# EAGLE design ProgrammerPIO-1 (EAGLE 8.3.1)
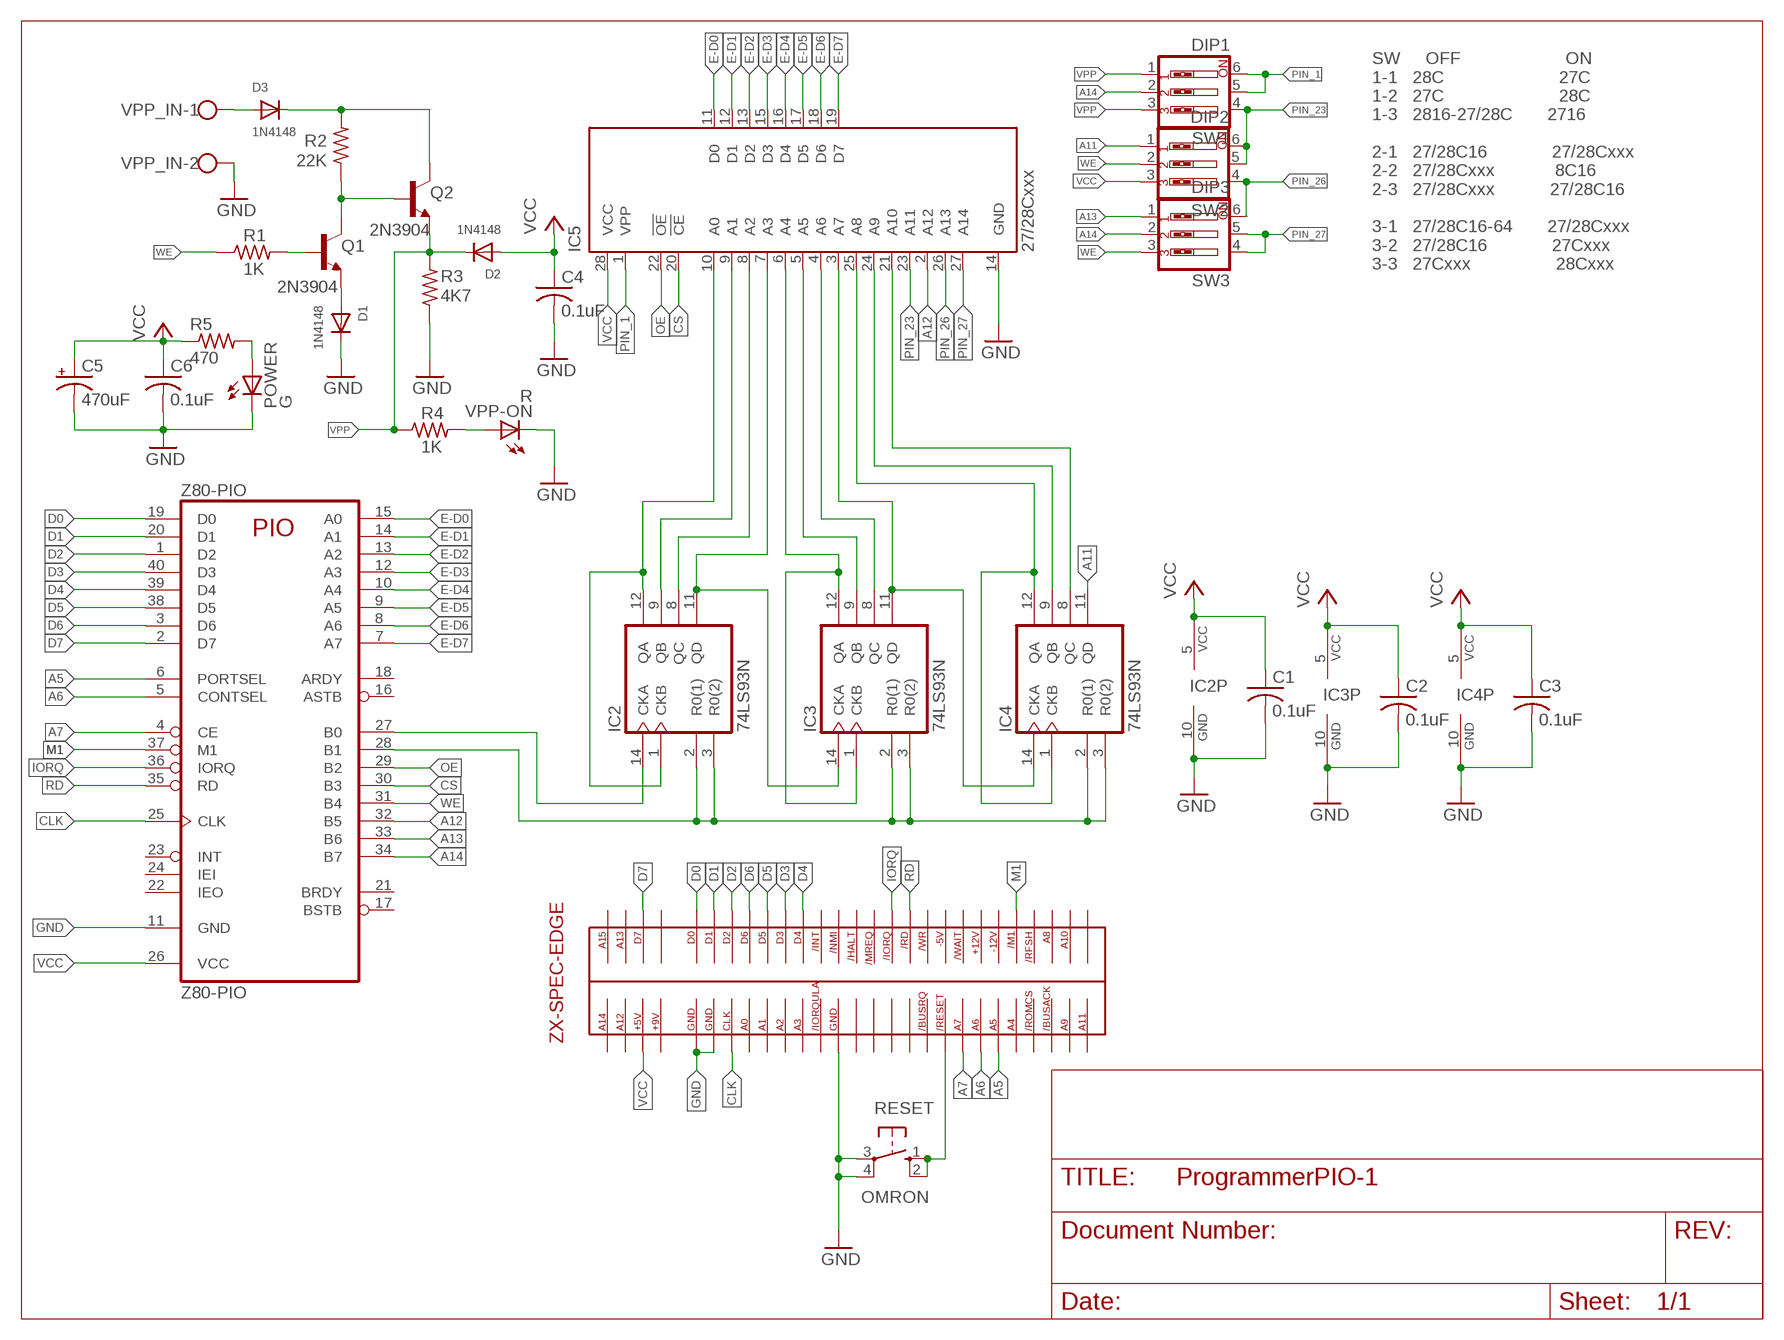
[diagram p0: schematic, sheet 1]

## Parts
1  ZX-EDGE-SPECCY  [ZX-EDGE-SPEC]
C1  0.1uF  C-US025-025X050  [C025-025X050]
C2  0.1uF  C-US025-025X050  [C025-025X050]
C3  0.1uF  C-US025-025X050  [C025-025X050]
C4  0.1uF  C-US025-025X050  [C025-025X050]
C5  470uF  CPOL-USE2.5-5  [E2,5-5]
C6  0.1uF  C-US025-025X050  [C025-025X050]
D1  1N4148  DIODEDO-1N4148  [DO-1N4148]
D2  1N4148  DIODEDO-1N4148  [DO-1N4148]
D3  1N4148  DIODEDO-1N4148  [DO-1N4148]
IC2  74LS93N  [DIL14]
IC3  74LS93N  [DIL14]
IC4  74LS93N  [DIL14]
IC5  27/28Cxxx  27C256P  [DIL28-6]
POWER  G  LED5MM  [LED5MM]
Q1  2N3904  [TO92]
Q2  2N3904  [TO92]
R1  1K  R-US_0204/7  [0204/7]
R2  22K  R-US_0204/7  [0204/7]
R3  4K7  R-US_0204/7  [0204/7]
R4  1K  R-US_0204/7  [0204/7]
R5  470  R-US_0204/7  [0204/7]
RESET  OMRON  10-XX  [B3F-10XX]
SW1  DIP1  SW_DIP-3  [EDG-03]
SW2  DIP2  SW_DIP-3  [EDG-03]
SW3  DIP3  SW_DIP-3  [EDG-03]
VPP-ON  R  LED5MM  [LED5MM]
VPP_IN  W237-102  [W237-102]
Z80-PIO  Z80-PIO  Z80PIO  [DIL40]

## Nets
A5: 1.A5 Z80-PIO.6(PORTSEL)
A6: 1.A6 Z80-PIO.5(CONTSEL)
A7: 1.A7 Z80-PIO.4(CE)
A11: IC4.11(QD) SW2.1
A12: IC5.2(A12) Z80-PIO.32(B5)
A13: SW3.1 Z80-PIO.33(B6)
A14: SW1.2 SW3.2 Z80-PIO.34(B7)
B0: IC2.14(CKA) Z80-PIO.27(B0)
B1: IC2.2(R0(1)) IC2.3(R0(2)) IC3.2(R0(1)) IC3.3(R0(2)) IC4.2(R0(1)) IC4.3(R0(2)) Z80-PIO.28(B1)
CLK: 1.CLK Z80-PIO.25(CLK)
CS: IC5.20(!CE) Z80-PIO.30(B3)
D0: 1.D0 Z80-PIO.19(D0)
D1: 1.D1 Z80-PIO.20(D1)
D2: 1.D2 Z80-PIO.1(D2)
D3: 1.D3 Z80-PIO.40(D3)
D4: 1.D4 Z80-PIO.39(D4)
D5: 1.D5 Z80-PIO.38(D5)
D6: 1.D6 Z80-PIO.3(D6)
D7: 1.D7 Z80-PIO.2(D7)
E-D0: IC5.11(D0) Z80-PIO.15(A0)
E-D1: IC5.12(D1) Z80-PIO.14(A1)
E-D2: IC5.13(D2) Z80-PIO.13(A2)
E-D3: IC5.15(D3) Z80-PIO.12(A3)
E-D4: IC5.16(D4) Z80-PIO.10(A4)
E-D5: IC5.17(D5) Z80-PIO.9(A5)
E-D6: IC5.18(D6) Z80-PIO.8(A6)
E-D7: IC5.19(D7) Z80-PIO.7(A7)
GND: 1.GND1 1.GND2 1.GND3 C1.2 C2.2 C3.2 C4.2 C5.- C6.2 D1.C IC2.10(GND) IC3.10(GND) IC4.10(GND) IC5.14(GND) POWER.K(C) R3.1 RESET.3(P) RESET.4(P1) VPP-ON.K(C) VPP_IN.2 Z80-PIO.11(GND)
IORQ: 1./IORQ Z80-PIO.36(IORQ)
M1: 1./M1 Z80-PIO.37(M1)
N$1: IC2.1(CKB) IC2.12(QA) IC5.10(A0)
N$2: IC2.9(QB) IC5.9(A1)
N$3: IC2.8(QC) IC5.8(A2)
N$4: IC2.11(QD) IC3.14(CKA) IC5.7(A3)
N$5: IC3.1(CKB) IC3.12(QA) IC5.6(A4)
N$6: IC3.9(QB) IC5.5(A5)
N$7: IC3.8(QC) IC5.4(A6)
N$8: IC3.11(QD) IC4.14(CKA) IC5.3(A7)
N$9: IC4.1(CKB) IC4.12(QA) IC5.25(A8)
N$10: IC4.9(QB) IC5.24(A9)
N$11: IC4.8(QC) IC5.21(A10)
N$13: Q1.2(B) R1.2
N$14: D1.A Q1.3(E)
N$15: Q1.1(C) Q2.2(B) R2.1
N$16: D3.A VPP_IN.1
N$17: D3.C Q2.1(C) R2.2
N$18: R4.2 VPP-ON.A
N$19: 1./RST RESET.1(S) RESET.2(S1)
N$20: POWER.A R5.2
OE: IC5.22(!OE) Z80-PIO.29(B2)
PIN_1: IC5.1(VPP) SW1.5 SW1.6
PIN_23: IC5.23(A11) SW1.4 SW2.5 SW2.6
PIN_26: IC5.26(A13) SW2.4 SW3.6
PIN_27: IC5.27(A14) SW3.4 SW3.5
RD: 1./RD Z80-PIO.35(RD)
VCC: 1.+5 C1.1 C2.1 C3.1 C4.1 C5.+ C6.1 D2.A IC2.5(VCC) IC3.5(VCC) IC4.5(VCC) IC5.28(VCC) R5.1 SW2.3 Z80-PIO.26(VCC)
VPP: D2.C Q2.3(E) R3.2 R4.1 SW1.1 SW1.3
WE: R1.1 SW2.2 SW3.3 Z80-PIO.31(B4)
Unconnected: 1.+9 1.+12 1.-5(-5V) 1.-12 1./BUSAK 1./BUSRQ 1./HALT 1./INT 1./IORQULA 1./MREQ 1./NMI 1./RFSH(/REFSH) 1./ROMCS 1./WAIT 1./WR 1.A0 1.A1 1.A2 1.A3 1.A4 1.A8 1.A9 1.A10 1.A11 1.A12 1.A13 1.A14 1.A15 1.N/C1 1.N/C2 1.N/C3 1.N/C4 1.N/C5 1.N/C6 Z80-PIO.16(ASTB) Z80-PIO.17(BSTB) Z80-PIO.18(ARDY) Z80-PIO.21(BRDY) Z80-PIO.22(IEO) Z80-PIO.23(INT) Z80-PIO.24(IEI)

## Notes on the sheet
- SW     OFF                     ON
  1-1   28C                       27C
  1-2   27C                       28C
  1-3   2816-27/28C       2716
  
  2-1   27/28C16             27/28Cxxx
  2-2   27/28Cxxx            8C16
  2-3   27/28Cxxx           27/28C16
  
  3-1   27/28C16-64       27/28Cxxx
  3-2   27/28C16             27Cxxx
  3-3   27Cxxx                 28Cxxx

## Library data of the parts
1 = sinclair-zx-spec:ZX-EDGE-SPECCY: ZX SPECTRUM EDGE CONNECTOR
C1-C4 C6 = rcl:C-US: CAPACITOR, American symbol
C5 = rcl:CPOL-US: POLARIZED CAPACITOR, American symbol
D1-D3 = adafruit:DIODE: Diode
IC2-IC4 = 74xx-us:74*93: Decade, divide by twelve and binary COUNTER
IC5 = microchip:27*256: CMOS EPROM 256 K (32 K x 8), low voltage; MF: Arrow Electronics; MPN: M27C256B15F1; OC_FARNELL: 1125431; OC_NEWARK: 93K7335
POWER = adafruit:LED: LED
Q1 Q2 = transistor-npn:2N3904: NPN Transistor
R1-R5 = rcl:R-US_: RESISTOR, American symbol
RESET = switch-omron:10-XX: OMRON SWITCH; MPN: B3F-1000; OC_FARNELL: 176432; OC_NEWARK: 36M3542
SW1-SW3 = special:SW_DIP-3: DIP SWITCH
VPP-ON = led:LED: LED
VPP_IN = con-wago-500:W237-102: WAGO SCREW CLAMP; MPN: 237-102; OC_FARNELL: unknown; OC_NEWARK: 70K9898
Z80-PIO = zilog:Z80PIO: Z80 FAMILY DEVICE

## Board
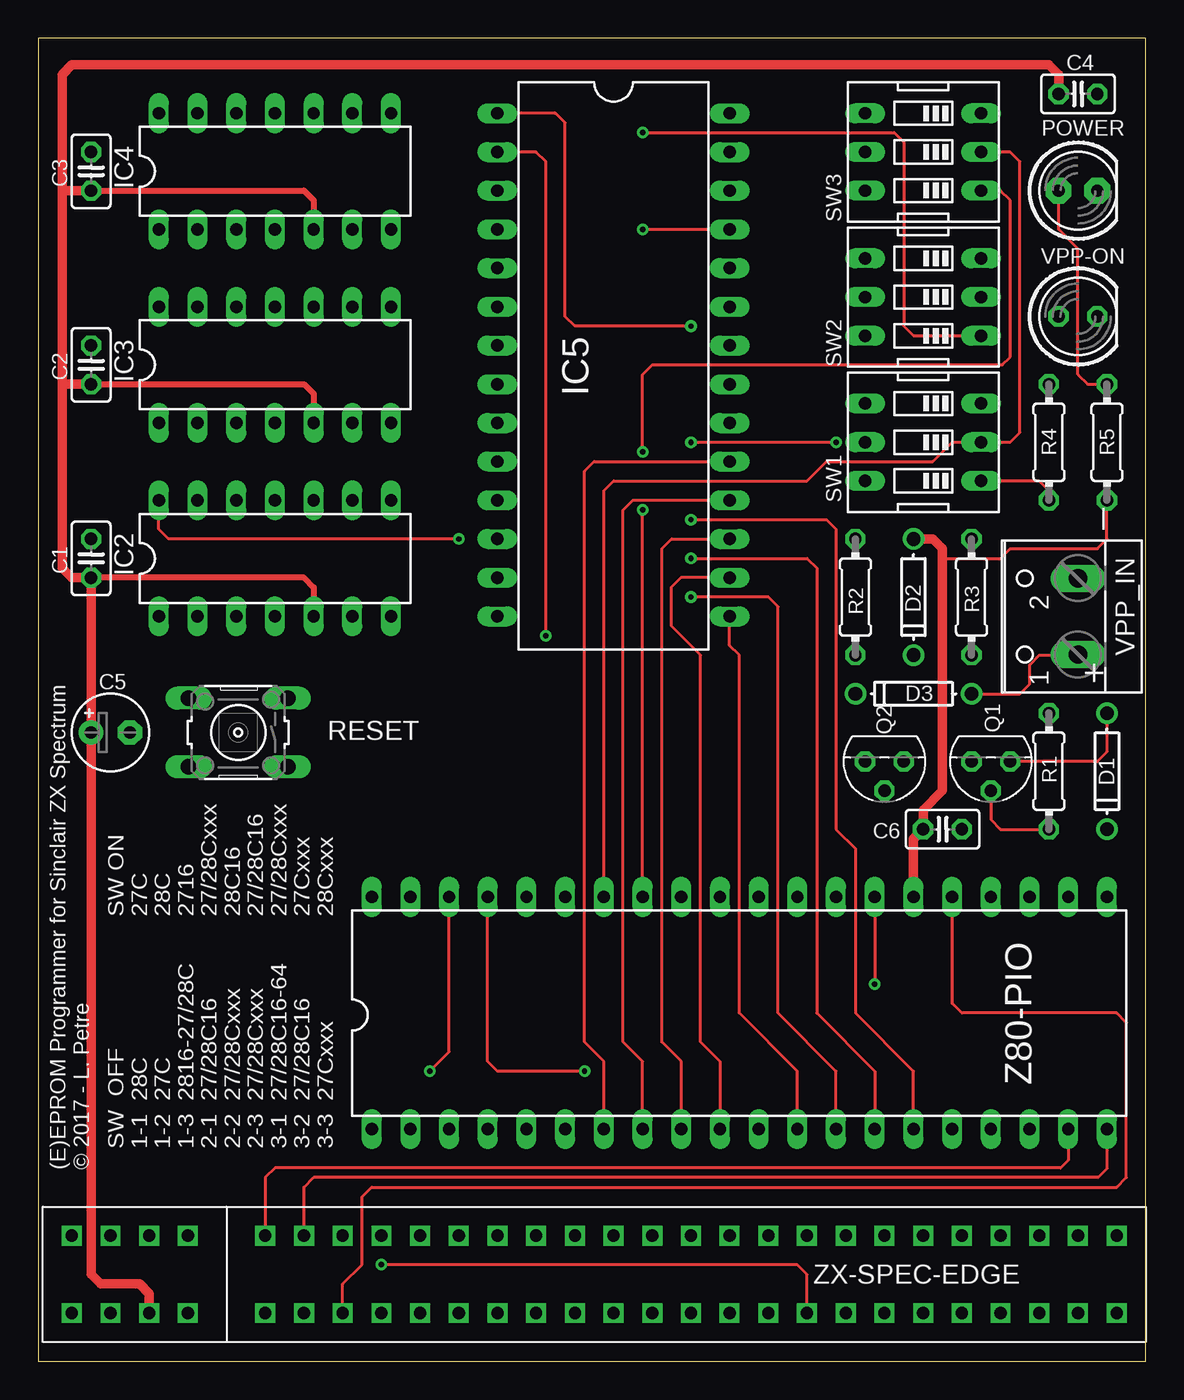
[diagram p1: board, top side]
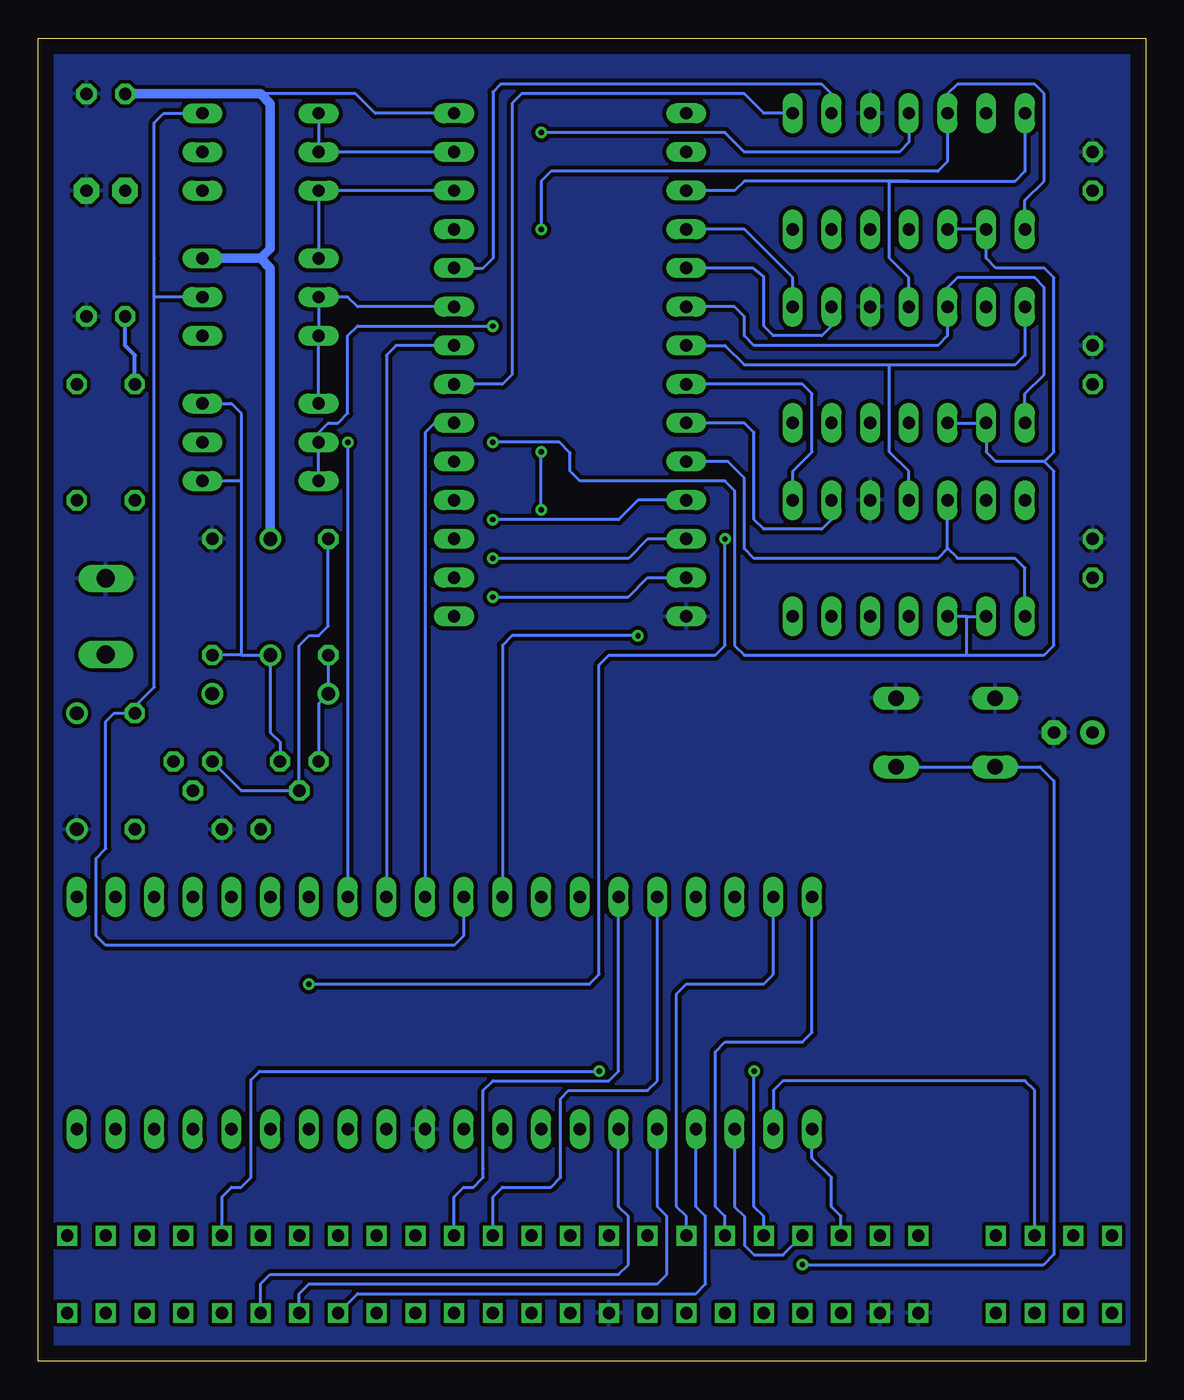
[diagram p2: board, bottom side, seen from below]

Size 72.7 x 86.85 mm. Coordinates in mm from the lower left corner, seen from the top.
Outline: 72.7,0 72.7,86.85 0,86.85 0,0 72.7,0
Copper layers (1*16): Top 0.035mm / dielectric 1.5mm / Bottom 0.035mm
Design rules "default": minimum track width 6mil, minimum drill 0.35mm, track to track 6mil, track to pad 6mil, pad to pad 6mil, via to via 6mil, smd to smd 6mil, copper to edge 40mil, drill to drill 6mil, minimum pad ring 10mil, minimum via ring 8mil, stop-mask expansion 4mil, vias tented up to drill 0mil, thermal gap 10mil

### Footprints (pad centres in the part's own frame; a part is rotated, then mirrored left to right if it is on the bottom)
ZX-EDGE-SPEC = drill 0.8 square: +5 -5.08,-2.54; +9 -2.54,-2.54; +12 43.18,2.54; -5 38.1,2.54; -12 45.72,2.54; /BUSAK 53.34,-2.54; /BUSRQ 35.56,-2.54; /HALT 25.4,2.54; /INT 20.32,2.54; /IORQ 30.48,2.54; /IORQULA 20.32,-2.54; /M1 48.26,2.54; /MREQ 27.94,2.54; /NMI 22.86,2.54; /RD 33.02,2.54; /RFSH 50.8,2.54; /ROMCS 50.8,-2.54; /RST 38.1,-2.54; /WAIT 40.64,2.54; /WR 35.56,2.54; A0 10.16,-2.54; A1 12.7,-2.54; A2 15.24,-2.54; A3 17.78,-2.54; A4 48.26,-2.54; A5 45.72,-2.54; A6 43.18,-2.54; A7 40.64,-2.54; A8 53.34,2.54; A9 55.88,-2.54; A10 55.88,2.54; A11 58.42,-2.54; A12 -7.62,-2.54; A13 -7.62,2.54; A14 -10.16,-2.54; A15 -10.16,2.54; CLK 7.62,-2.54; D0 2.54,2.54; D1 5.08,2.54; D2 7.62,2.54; D3 15.24,2.54; D4 17.78,2.54; D5 12.7,2.54; D6 10.16,2.54; D7 -5.08,2.54; GND1 2.54,-2.54; GND2 5.08,-2.54; GND3 22.86,-2.54; N/C1 -2.54,2.54; N/C2 58.42,2.54; N/C3 25.4,-2.54; N/C4 27.94,-2.54; N/C5 30.48,-2.54; N/C6 33.02,-2.54
C025-025X050 = drill 0.813 octagon: 1 -1.27,0; 2 1.27,0
E2,5-5 = drill 0.813 pad 1.6: + -1.27,0 | drill 0.813 pad 1.6 octagon: - 1.27,0
DO-1N4148 = drill 0.9: A -3.81,0; C 3.81,0
DIL14 = drill 0.813 long: 1 -7.62,-3.81; 2 -5.08,-3.81; 3 -2.54,-3.81; 4 0,-3.81; 5 2.54,-3.81; 6 5.08,-3.81; 7 7.62,-3.81; 8 7.62,3.81; 9 5.08,3.81; 10 2.54,3.81; 11 0,3.81; 12 -2.54,3.81; 13 -5.08,3.81; 14 -7.62,3.81
DIL28-6 = drill 0.813 long: 1 -16.51,-7.62; 2 -13.97,-7.62; 3 -11.43,-7.62; 4 -8.89,-7.62; 5 -6.35,-7.62; 6 -3.81,-7.62; 7 -1.27,-7.62; 8 1.27,-7.62; 9 3.81,-7.62; 10 6.35,-7.62; 11 8.89,-7.62; 12 11.43,-7.62; 13 13.97,-7.62; 14 16.51,-7.62; 15 16.51,7.62; 16 13.97,7.62; 17 11.43,7.62; 18 8.89,7.62; 19 6.35,7.62; 20 3.81,7.62; 21 1.27,7.62; 22 -1.27,7.62; 23 -3.81,7.62; 24 -6.35,7.62; 25 -8.89,7.62; 26 -11.43,7.62; 27 -13.97,7.62; 28 -16.51,7.62
LED5MM = drill 0.813 pad 1.676 octagon: A -1.27,0; K 1.27,0
TO92 = drill 0.813 octagon: 1 1.27,0; 2 0,1.905; 3 -1.27,0
0204/7 = drill 0.813 octagon: 1 -3.81,0; 2 3.81,0
B3F-10XX = drill 1.016 long: 1 -3.251,2.261; 2 3.251,2.261; 3 -3.251,-2.261; 4 3.251,-2.261
EDG-03 = drill 0.813 long: 1 -2.54,-3.81; 2 0,-3.81; 3 2.54,-3.81; 4 2.54,3.81; 5 0,3.81; 6 -2.54,3.81
LED5MM' = drill 0.813 octagon: A -1.27,0; K 1.27,0
W237-102 = drill 1.194 long: 1 -2.5,-1.27; 2 2.5,-1.27
DIL40 = drill 0.813 long: 1 -24.13,-7.62; 2 -21.59,-7.62; 3 -19.05,-7.62; 4 -16.51,-7.62; 5 -13.97,-7.62; 6 -11.43,-7.62; 7 -8.89,-7.62; 8 -6.35,-7.62; 9 -3.81,-7.62; 10 -1.27,-7.62; 11 1.27,-7.62; 12 3.81,-7.62; 13 6.35,-7.62; 14 8.89,-7.62; 15 11.43,-7.62; 16 13.97,-7.62; 17 16.51,-7.62; 18 19.05,-7.62; 19 21.59,-7.62; 20 24.13,-7.62; 21 24.13,7.62; 22 21.59,7.62; 23 19.05,7.62; 24 16.51,7.62; 25 13.97,7.62; 26 11.43,7.62; 27 8.89,7.62; 28 6.35,7.62; 29 3.81,7.62; 30 1.27,7.62; 31 -1.27,7.62; 32 -3.81,7.62; 33 -6.35,7.62; 34 -8.89,7.62; 35 -11.43,7.62; 36 -13.97,7.62; 37 -16.51,7.62; 38 -19.05,7.62; 39 -21.59,7.62; 40 -24.13,7.62

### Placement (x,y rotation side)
1  12.37,5.71 0 top
C1  3.48,52.7 90 top
C2  3.48,65.41 90 top
C3  3.48,78.11 90 top
C4  68.25,83.19 0 top
C5  4.75,41.27 0 top
C6  59.36,34.92 0 top
D1  70.16,38.73 270 top
D2  57.45,50.16 270 top
D3  57.45,43.81 180 top
IC2  15.54,52.7 0 top
IC3  15.54,65.41 0 top
IC4  15.54,78.11 0 top
IC5  37.77,65.41 270 top
POWER  68.25,76.83 0 top
Q1  62.54,39.37 180 top
Q2  55.55,39.37 180 top
R1  66.34,38.73 270 top
R2  53.65,50.16 270 top
R3  61.27,50.16 270 top
R4  66.34,60.33 90 top
R5  70.16,60.33 90 top
RESET  13.13,41.27 180 top
SW1  58.09,60.33 90 top
SW2  58.09,69.85 90 top
SW3  58.09,79.38 90 top
VPP-ON  R  [LED5MM']  68.25,68.58 0 top
VPP_IN  66.98,48.9 90 top
Z80-PIO  46.02,22.86 0 top

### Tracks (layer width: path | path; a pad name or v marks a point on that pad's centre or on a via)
A5
  Bottom 0.2: 1.A5 58.09,5.08 57.45,5.71 34.59,5.71 33.96,6.35 33.96,9.53 34.59,10.16 Z80-PIO.6
A6
  Bottom 0.2: 1.A6 55.55,4.45 54.91,5.08 32.05,5.08 31.42,5.71 31.42,9.53 32.05,10.16 Z80-PIO.5
A7
  Bottom 0.2: 1.A7 51.74,4.45 29.52,4.45 28.88,5.08 28.88,9.53 29.52,10.16 Z80-PIO.4
A11  (via drill 0.35)
  Top 0.2: v39.68,80.64 56.19,80.64 56.82,80.01 56.82,67.94 57.45,67.31 SW2.1
  Bottom 0.2: IC4.11 15.54,80.01 16.18,79.38 26.34,79.38 27.61,80.64 v39.68,80.64
A12  (via drill 0.35)
  Top 0.2: v33.33,47.62 33.33,78.74 32.69,79.38 IC5.2
  Bottom 0.2: v33.33,47.62 41.58,47.62 42.22,46.99 Z80-PIO.32
A13  (via drill 0.35)
  Top 0.2: SW3.1 63.17,76.83 63.81,76.2 63.81,65.91 63.3,65.41 40.31,65.41 39.68,64.77 v39.68,59.69 | Z80-PIO.33 v39.68,55.88
  Bottom 0.2: v39.68,55.88 v39.68,59.69
A14
  Top 0.2: Z80-PIO.34 37.14,57.15 37.77,57.78 50.47,57.78 51.74,59.05 58.73,59.05 60,60.33 SW1.2 63.81,60.33 64.44,60.96 64.44,78.74 63.81,79.38 SW3.2
B0  (via drill 0.35)
  Top 0.2: Z80-PIO.27 v54.91,24.77 | v27.61,53.98 8.56,53.98 7.93,54.61 IC2.14
  Bottom 0.2: v54.91,24.77 36.5,24.77 35.87,25.4 35.87,45.72 35.23,46.35 28.25,46.35 27.61,46.99 v27.61,53.98
B1  (via drill 0.35)
  Top 0.2: v42.85,60.33 v52.38,60.33
  Bottom 0.2: 11.76,48.9 IC2.2 | 11.76,48.9 IC2.3 | IC3.3 IC3.2 10.46,59.69 9.83,59.05 6.66,59.05 | IC4.3 IC4.2 10.46,72.39 9.83,71.75 6.66,71.75 6.02,71.12 6.02,59.69 6.66,59.05 | 11.73,46.35 6.66,46.35 6.02,46.99 6.02,58.42 6.66,59.05 | v52.38,60.33 Z80-PIO.28 | v42.85,60.33 38.47,60.33 37.77,59.62 37.77,58.42 37.14,57.78 27.61,57.78 26.98,57.15 26.98,46.99 26.34,46.35 11.73,46.35 | 11.73,46.35 11.73,48.87 11.76,48.9
CLK
  Top 0.2: 1.CLK 19.99,5.08 21.26,6.35 21.26,10.79 21.9,11.43 70.79,11.43 71.42,12.06 71.42,22.23 70.79,22.86 60.63,22.86 60,23.5 Z80-PIO.25
CS
  Bottom 0.2: IC5.20 46.66,61.59 47.3,60.96 Z80-PIO.30
D0
  Top 0.2: 1.D0 14.91,12.06 15.54,12.7 67.11,12.7 67.61,13.21 Z80-PIO.19
D1
  Top 0.2: 1.D1 17.45,11.43 18.09,12.06 69.57,12.06 70.16,12.65 Z80-PIO.20
D2
  Bottom 0.2: 1.D2 19.99,9.53 20.62,10.16 20.62,12.06 21.9,13.34 Z80-PIO.1
D3
  Bottom 0.2: 1.D3 27.61,9.53 28.25,10.16 28.25,20.32 27.61,20.95 22.53,20.95 21.9,21.59 Z80-PIO.40
D4
  Bottom 0.2: 1.D4 30.15,9.53 30.79,10.16 30.79,24.13 30.15,24.77 25.07,24.77 24.44,25.4 Z80-PIO.39
D5  (via drill 0.35)
  Top 0.2: v25.71,19.05 26.98,20.32 Z80-PIO.38
  Bottom 0.2: 1.D5 25.07,9.53 25.71,10.16 v25.71,19.05
D6
  Bottom 0.2: Z80-PIO.3 26.98,10.16 26.34,9.53 26.34,7.62 25.71,6.99 23.8,6.99 1.D6
D7
  Bottom 0.2: 1.D7 7.29,17.78 7.93,18.41 23.8,18.41 24.44,17.78 Z80-PIO.2
E-D0  (via drill 0.35)
  Top 0.2: Z80-PIO.15 57.45,19.05 53.65,22.86 53.65,33.66 52.38,34.92 52.38,54.61 51.74,55.24 v42.85,55.24
  Bottom 0.2: IC5.11 33.33,56.52 34.59,55.24 v42.85,55.24
E-D1  (via drill 0.35)
  Top 0.2: v42.85,52.7 50.47,52.7 51.11,52.07 51.11,22.86 54.91,19.05 Z80-PIO.14
  Bottom 0.2: IC5.12 32.69,53.98 33.96,52.7 v42.85,52.7
E-D2  (via drill 0.35)
  Top 0.2: Z80-PIO.13 52.38,19.05 48.57,22.86 48.57,49.53 47.93,50.16 v42.85,50.16
  Bottom 0.2: v42.85,50.16 33.96,50.16 32.69,51.44 IC5.13
E-D3
  Top 0.2: IC5.15 45.39,46.99 46.02,46.35 46.02,22.86 49.84,19.05 Z80-PIO.12
E-D4
  Top 0.2: Z80-PIO.10 44.76,19.68 43.48,20.95 43.48,46.35 41.58,48.26 41.58,50.83 42.18,51.44 IC5.16
E-D5
  Top 0.2: Z80-PIO.9 42.22,19.68 40.95,20.95 40.95,53.34 41.58,53.98 IC5.17
E-D6
  Top 0.2: Z80-PIO.8 39.68,19.68 38.41,20.95 38.41,55.88 39.04,56.52 IC5.18
E-D7
  Top 0.2: Z80-PIO.7 37.14,19.68 35.87,20.95 35.87,58.42 36.5,59.05 IC5.19
GND
  pour Bottom (isolate 0.254): 72.7,0 0.05,-0.13 0.05,86.87 72.82,86.87 72.57,0.13
IORQ
  Bottom 0.2: 1./IORQ 42.85,10.79 42.22,11.43 39.04,11.43 38.41,12.06 38.41,17.25 37.87,17.78 32.69,17.78 32.05,18.41 Z80-PIO.36
M1  (via drill 0.35)
  Top 0.2: v35.87,19.05 30.15,19.05 29.52,19.68 Z80-PIO.37
  Bottom 0.2: 1./M1 60.63,10.79 60,11.43 59.36,11.43 58.73,12.06 58.73,18.49 58.16,19.05 v35.87,19.05
N$1
  Bottom 0.2: IC5.10 27.41,59.05 26.34,57.98 26.34,53.34 25.71,52.7 13.64,52.7 13.01,53.34 13.01,53.39 | 13.01,53.39 IC2.12 | IC2.1 7.93,52.07 8.56,52.7 12.37,52.7 12.37,52.75 13.01,53.39
N$2
  Bottom 0.2: IC2.9 20.62,55.24 21.26,54.61 25.07,54.61 25.71,55.24 25.71,60.96 26.34,61.59 IC5.9
N$3
  Bottom 0.2: IC2.8 23.17,58.42 21.9,59.69 21.9,63.5 22.53,64.14 IC5.8
N$4
  Bottom 0.2: IC3.14 7.93,66.04 8.56,65.41 16.91,65.41 | IC5.7 27.61,66.67 26.34,65.41 16.91,65.41 | IC2.11 15.54,58.42 16.82,59.69 16.82,65.31 16.91,65.41
N$5
  Bottom 0.2: IC3.1 7.93,63.5 6.66,64.77 6.66,70.48 7.29,71.12 12.37,71.12 13.01,70.48 IC3.12 13.01,67.31 13.64,66.67 25.71,66.67 26.34,67.31 26.34,68.58 26.98,69.22 IC5.6
N$6
  Bottom 0.2: IC3.9 20.62,67.94 21.26,67.31 24.44,67.31 25.07,67.94 25.07,71.19 25.76,71.75 IC5.5
N$7
  Bottom 0.2: IC3.8 23.17,71.12 26.34,74.3 IC5.4
N$8
  Bottom 0.2: IC4.14 7.93,78.11 8.56,77.47 15.55,77.47 | 15.55,77.47 26.34,77.47 26.98,76.83 IC5.3 | IC3.11 15.54,71.12 16.82,72.39 16.82,77.47 15.55,77.47
N$9  (via drill 0.35)
  Top 0.2: v39.68,74.3 IC5.25
  Bottom 0.2: IC4.1 7.93,76.2 6.66,77.47 6.66,83.19 7.29,83.82 12.37,83.82 13.01,83.19 IC4.12 13.01,78.74 13.64,78.11 39.04,78.11 39.68,77.47 v39.68,74.3
N$10
  Bottom 0.2: IC5.24 43.48,71.75 42.85,72.39 42.85,83.31 42.34,83.82 21.26,83.82 20.62,83.19 IC4.9
N$11
  Bottom 0.2: IC5.21 42.22,64.14 41.58,64.77 41.58,82.57 40.97,83.19 26.34,83.19 25.07,81.92 IC4.8
N$13
  Top 0.2: Q1.2 62.54,35.56 63.17,34.92 R1.2
N$14
  Top 0.2: D1.A 70.16,40.01 69.52,39.37 Q1.3
N$15
  Bottom 0.2: Q1.1 59.36,37.47 Q2.2 55.55,46.99 54.91,47.62 54.28,47.62 53.65,48.26 R2.1
N$16
  Top 0.2: D3.A 64.44,43.81 65.08,44.45 65.08,45.72 65.71,46.35 68.21,46.35 VPP_IN.1
N$17
  Bottom 0.2: R2.2 D3.C 54.28,43.18 Q2.1
N$18
  Bottom 0.254: R4.2 66.34,66.04 66.98,66.67 VPP-ON.A
N$19  (via drill 0.35)
  Top 0.2: 1./RST 50.47,5.71 49.84,6.35 v22.53,6.35
  Bottom 0.2: RESET.1 RESET.2 6.93,39.01 6.02,38.1 6.02,7.02 6.69,6.35 v22.53,6.35
N$20
  Top 0.2: POWER.A 66.98,74.3 68.25,73.03 68.25,64.77 68.89,64.14 R5.2
OE
  Bottom 0.2: IC5.22 49.2,66.67 49.84,66.04 Z80-PIO.29
PIN_1  (via drill 0.35)
  Top 0.2: v42.85,67.94 35.23,67.94 34.59,68.58 34.59,81.28 33.96,81.92 IC5.1
  Bottom 0.2: SW1.6 SW1.5 54.28,60.96 53.65,61.59 53.01,61.59 52.38,62.23 52.38,67.31 51.74,67.94 v42.85,67.94
PIN_23
  Bottom 0.2: SW1.4 SW2.6 SW2.5 52.38,69.85 51.74,69.22 IC5.23
PIN_26
  Bottom 0.2: IC5.26 SW3.6 SW2.4
PIN_27
  Bottom 0.2: IC5.27 54.22,79.38 54.28,79.43 | 54.28,79.43 SW3.5 | SW3.4 54.28,79.43
RD
  Bottom 0.2: 1./RD 45.39,10.79 44.76,11.43 44.12,11.43 43.48,12.06 43.48,12.66 43.5,12.68 43.48,12.7 43.48,17.78 42.85,18.41 35.23,18.41 34.59,19.05 Z80-PIO.35
VCC
  Top 0.2: 59.52,52.07 59.36,51.91 | 59.36,52.7 59.36,52.71 63.17,52.71 63.81,53.34 69.52,53.34 70.16,53.98 R5.1
  Top 0.406: C1.1 17.45,51.44 18.09,50.8 IC2.5 | C2.1 17.45,64.14 18.09,63.5 IC3.5 | C3.1 17.45,76.83 18.09,76.2 IC4.5
  Top 0.61: Z80-PIO.26 57.45,34.29 C6.1 58.09,36.2 59.36,37.47 59.36,51.91 59.36,52.71 59.36,53.34 58.73,53.98 D2.A | 1.+5 7.29,4.45 6.66,5.08 4.12,5.08 3.48,5.71 C5.+ C1.1 2.21,51.44 1.57,52.07 1.57,64.14 | 1.57,64.14 C2.1 | 1.57,64.14 1.57,76.83 | 1.57,76.83 C3.1 | 1.57,76.83 1.57,84.45 2.21,85.09 66.34,85.09 66.98,84.45 C4.1
  Bottom 0.2: 58.09,83.19 51.84,83.19 50.57,81.92 IC5.28
  Bottom 0.61: C4.1 58.09,83.19 57.45,82.55 57.45,73.03 58.09,72.39 | 58.09,72.39 SW2.3 | 58.09,72.39 57.45,71.75 D2.A
VPP
  Top 0.2: SW1.1 65.71,57.78 66.34,57.15 R4.1
  Bottom 0.2: SW1.3 60,62.87 59.36,62.23 59.36,57.78 | 59.36,57.78 SW1.1 | 59.36,57.78 59.36,46.35 | 59.36,46.35 R3.2 | 59.36,46.35 D2.C 57.45,41.27 56.82,40.64 Q2.3
WE
  Bottom 0.2: 63.17,81.92 SW3.3 64.44,81.92 65.08,81.28 65.08,72.4 | Z80-PIO.31 44.76,27.94 45.39,27.3 68.25,27.3 68.89,27.94 68.89,33.02 68.25,33.66 68.25,41.99 67.7,42.55 R1.1 66.34,42.98 65.08,44.25 65.08,72.4 | SW2.2 65.06,69.85 65.08,72.4

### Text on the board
tNames: _ | + | SW ON / 27C / 28C / 2716 / 27/28Cxxx / 28C16 / 27/28C16 / 27/28Cxxx / 27Cxxx / 28Cxxx | SW OFF / 1-1 28C / 1-2 27C / 1-3 2816-27/28C / 2-1 27/28C16 / 2-2 27/28Cxxx / 2-3 27/28Cxxx / 3-1 27/28C16-64 / 3-2 27/28C16 / 3-3 27Cxxx | (E)EPROM Programmer for Sinclair ZX Spectrum / © 2017 - L. Petre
